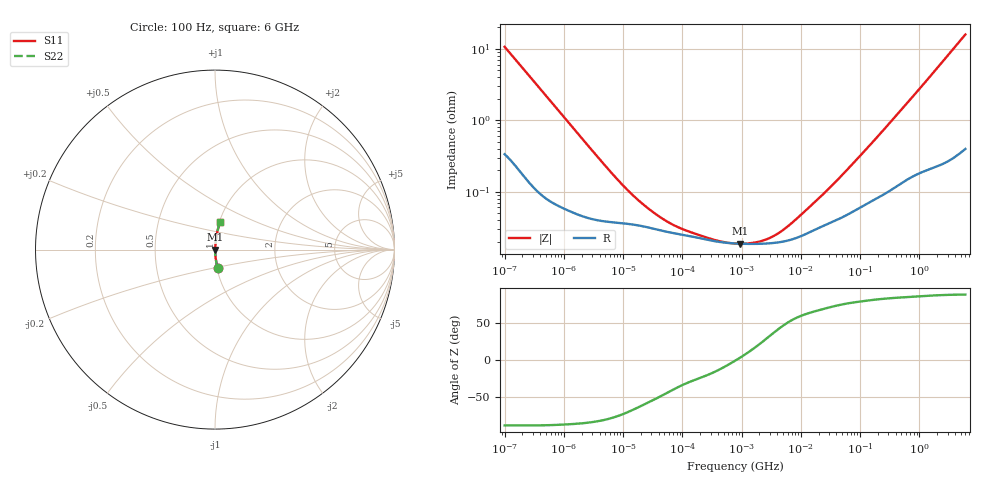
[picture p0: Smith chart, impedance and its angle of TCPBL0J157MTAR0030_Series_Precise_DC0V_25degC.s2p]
! TCPBL0J157MTAR0030 Polymer Tantalum Capacitor Sparameter Model
! Model Generated by Samsung Electro-Mechanics
! Samsung Sparameter Version 5.0
! Date : Oct-21-2025
! Products : Polymer Tantalum Capacitor
! Characteristics :
!  Nominal Capacitance = 150uF
!  Capacitance Tolerance = +/-20%
!  ESR = 30 mohm max at 100kHz
!  Rated Voltage = 6.3Vdc
!  Size = 1411(unit:inch), 3528(unit:mm)
!  Length = 3.50+/-0.20mm
!  Width = 2.80+/-0.20mm
!  Thickness = 1.1+/-0.10mm
!  Lineup = Conductive Polymer Type
!  Feature = PBL
!  Measurement Temperature : 25degC.
!  DC bias Value = 0V
!  Frequency : 100Hz ~ 6GHz
! External Node Assignments :
!  1  o---||---o  2
# MHz S RI R 50.0
! Freq.  Real(S11)  Im(S11)  Real(S12)  Im(S12)  Real(S21)  Im(S21)  Real(S22)  Im(S22)
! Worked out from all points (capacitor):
!   300 points, 100 Hz to 6 GHz, reference 50 ohm
!   read as one part in series: C = 148 uF near 106.2 Hz
!   lowest |Z| = 18.7 mohm at 955.3 kHz (marker M1)
!   series resonance near 808.9 kHz, so ESL is about 260 pH
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0.0001  0.0145 -0.1047  0.9855 0.1047  0.9855 0.1047  0.0145 -0.1047
0.0001714451  0.00596 -0.0625  0.994 0.0625  0.994 0.0625  0.00596 -0.0625
0.0003313429  0.00215 -0.0328  0.9978 0.0328  0.9978 0.0328  0.00215 -0.0328
0.001998454  0.000487 -0.00559  0.9995 0.00559  0.9995 0.00559  0.000487 -0.00559
0.005874137  0.000379 -0.00194  0.9996 0.00194  0.9996 0.00194  0.000379 -0.00194
0.01135264  0.000356 -0.00103  0.9996 0.00103  0.9996 0.00103  0.000356 -0.00103
0.02066501  0.00033 -0.000605  0.9997 0.000605  0.9997 0.000605  0.00033 -0.000605
0.03993819  0.000291 -0.000347  0.9997 0.000347  0.9997 0.000347  0.000291 -0.000347
0.0726988  0.000261 -0.000213  0.9997 0.000213  0.9997 0.000213  0.000261 -0.000213
0.1405012  0.000236 -0.000129  0.9998 0.000129  0.9998 0.000129  0.000236 -0.000129
0.3889699  0.000199 -5.03e-05  0.9998 5.03e-05  0.9998 5.03e-05  0.000199 -5.03e-05
0.7981464  0.000187 -9.04e-07  0.9998 9.04e-07  0.9998 9.04e-07  0.000187 -9.04e-07
0.9552658  0.000186 1.16e-05  0.9998 -1.16e-05  0.9998 -1.16e-05  0.000186 1.16e-05
1.960157  0.000186 7.11e-05  0.9998 -7.11e-05  0.9998 -7.11e-05  0.000186 7.11e-05
3.56804  0.000191 0.000147  0.9998 -0.000147  0.9998 -0.000147  0.000191 0.000147
6.494841  0.00021 0.000272  0.9998 -0.000272  0.9998 -0.000272  0.00021 0.000272
15.95059  0.000284 0.000611  0.9997 -0.000611  0.9997 -0.000611  0.000284 0.000611
52.85115  0.000449 0.00174  0.9996 -0.00174  0.9996 -0.00174  0.000449 0.00174
318.7652  0.00111 0.00914  0.9989 -0.00914  0.9989 -0.00914  0.00111 0.00914
1922.593  0.00486 0.0512  0.9951 -0.0512  0.9951 -0.0512  0.00486 0.0512
3499.664  0.0114 0.0918  0.9886 -0.0918  0.9886 -0.0918  0.0114 0.0918
6000  0.0282 0.1536  0.9718 -0.1536  0.9718 -0.1536  0.0282 0.1536
